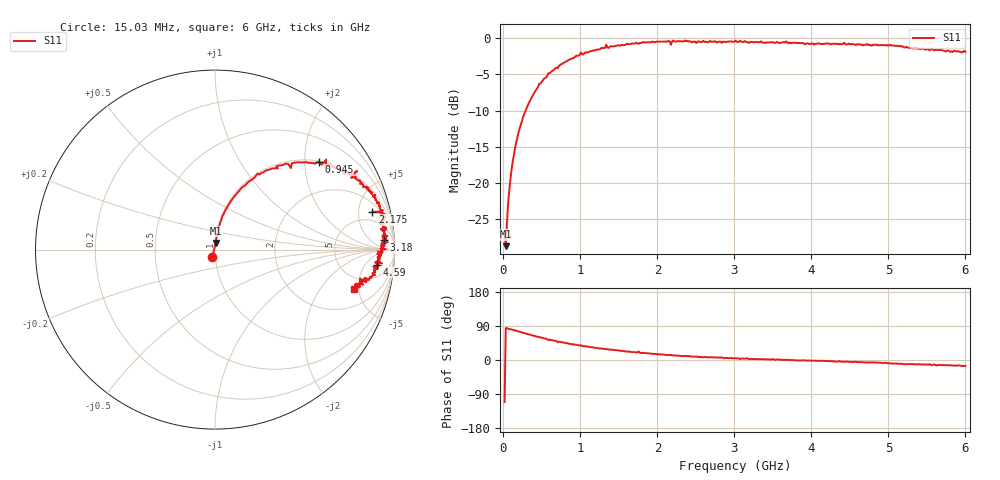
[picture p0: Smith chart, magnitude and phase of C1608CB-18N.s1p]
!	Network	Analyzer	HP8753E.07.74:	Oct	30	2002	Serial	No.	JP38451487
!	Hewlett-Packard
!	7	Sep	2009	9:38:10
!	Frequency	S11
#	HZ	S	RI	R	50
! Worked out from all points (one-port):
!   400 points, 15.03 MHz to 6 GHz, reference 50 ohm
!   lowest |S11| = -28.8 dB at 30.03 MHz (marker M1), VSWR 1.08, Z = 50.3 + j3.65 ohm
!   |S11| at or under -10 dB: start of sweep to 287.8 MHz
!   S11 on the Smith chart (normalised r, x): 15.03 MHz: 0.97, -0.08; 945 MHz: 1.02, +2.34; 2.175 GHz: 3.15, +7.09; 3.18 GHz: 18, +16; 4.59 GHz: 11, -10; 6 GHz: 3.59, -4.46
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1.502992e7  -0.016 -0.0422
3.002985e7  0.00387 0.0363
6.00297e7  0.00886 0.0709
1.050295e8  0.0207 0.121
1.650292e8  0.0409 0.186
2.550287e8  0.0891 0.271
4.650277e8  0.237 0.424
7.650262e8  0.455 0.485
9.450253e8  0.577 0.489
1.335023e9  0.792 0.438
1.365023e9  0.759 0.399
1.515022e9  0.808 0.366
1.725021e9  0.876 0.318
1.755021e9  0.845 0.35
1.785021e9  0.884 0.292
2.145019e9  0.936 0.219
2.175019e9  0.877 0.21
2.205019e9  0.945 0.199
2.265019e9  0.937 0.193
2.565017e9  0.935 0.118
2.835016e9  0.924 0.115
3.015015e9  0.961 0.0764
3.180014e9  0.94 0.0518
3.765011e9  0.929 -0.00354
4.515007e9  0.91 -0.0724
4.590007e9  0.903 -0.0833
5.265004e9  0.845 -0.166
6e9  0.776 -0.218
